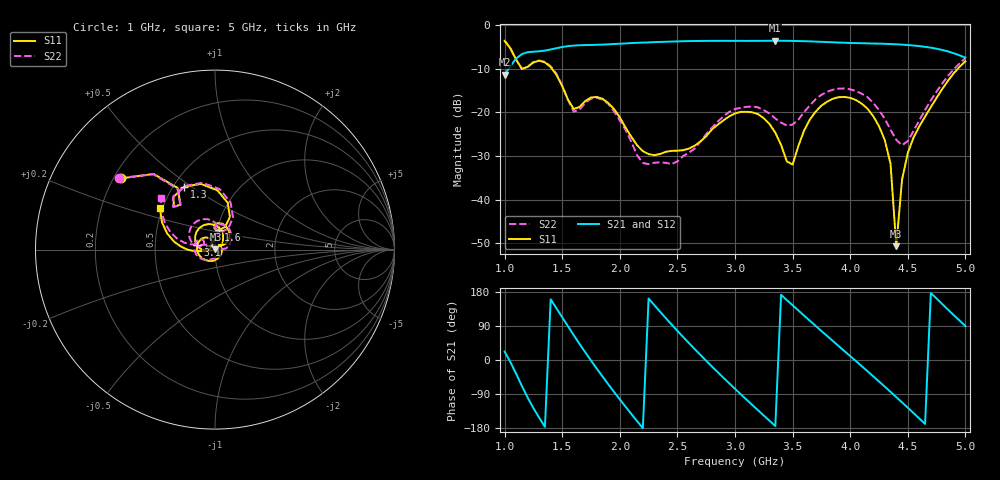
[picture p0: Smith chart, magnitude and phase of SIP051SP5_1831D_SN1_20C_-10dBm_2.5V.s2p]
# GHz  S  dB  R  50
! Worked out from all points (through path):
!   81 points, 1 GHz to 5 GHz, reference 50 ohm
!   highest |S21| = -3.59 dB at 3.35 GHz (marker M1); lowest = -11.4 dB at 1 GHz (marker M2)
!   lowest |S11| = -50.6 dB at 4.4 GHz (marker M3), VSWR 1.01, Z = 50.3 + j0.146 ohm
!   |S11| at or under -10 dB: 1.149433 GHz to 1.152709 GHz (3.276 MHz wide, 0.285 % of centre); 1.411 GHz to 4.935 GHz (3.524 GHz wide, 111 % of centre)
!   |S22| runs from -31.9 to -3.5 dB; largest |S21 - S12| = 0.0025
!   S11 on the Smith chart (normalised r, x): 1 GHz: 0.23, +0.32; 1.3 GHz: 0.57, +0.47; 1.6 GHz: 1.02, +0.22; 3.1 GHz: 0.82, +0.05; 5 GHz: 0.48, +0.26
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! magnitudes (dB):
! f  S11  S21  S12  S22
! 1 GHz  -3.6  -11.4  -11.4  -3.5
! 1.15 GHz  -10.0  -6.6  -6.6  -10.1
! 1.3 GHz  -8.2  -6.0  -6.0  -8.1
! 1.45 GHz  -11.4  -5.3  -5.3  -11.2
! 1.6 GHz  -19.2  -4.7  -4.7  -19.8
! 1.7 GHz  -17.4  -4.6  -4.6  -17.8
! 1.9 GHz  -17.9  -4.4  -4.4  -18.1
! 2.2 GHz  -28.9  -4.0  -4.0  -31.6
! 2.35 GHz  -29.5  -3.9  -3.9  -31.4
! 2.5 GHz  -28.8  -3.7  -3.7  -31.2
! 3 GHz  -20.2  -3.6  -3.6  -19.2
! 3.1 GHz  -19.9  -3.6  -3.6  -18.7
! 3.35 GHz  -24.7  -3.6  -3.6  -21.4
! 3.5 GHz  -31.9  -3.6  -3.6  -22.8
! 3.7 GHz  -19.8  -3.8  -3.8  -17.0
! 4.1 GHz  -18.0  -4.2  -4.1  -15.7
! 4.25 GHz  -23.1  -4.2  -4.2  -19.5
! 4.35 GHz  -31.7  -4.4  -4.3  -24.0
! 4.4 GHz  -50.6  -4.4  -4.4  -26.3
! 4.45 GHz  -35.4  -4.5  -4.5  -27.5
! 4.55 GHz  -25.8  -4.7  -4.7  -24.3
! 5 GHz  -8.3  -7.5  -7.5  -7.6
